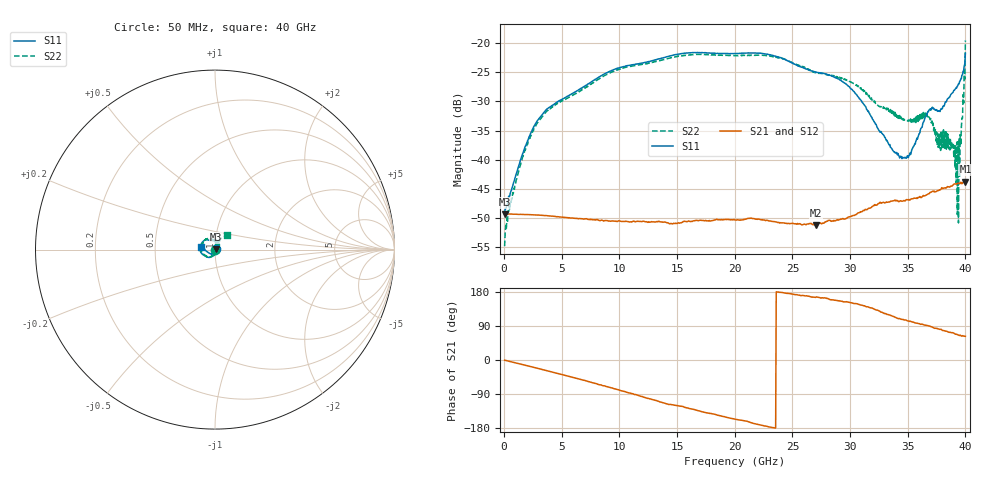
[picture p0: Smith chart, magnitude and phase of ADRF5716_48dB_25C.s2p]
! Device: ADRF5716
! Description: 30GHz 2-Bit Digital Attenuator
! Frequency: 100 MHz – 30 GHz
! Ports:
! ATTIN  = Port 1
! ATTOUT = Port 2
! State: 48 dB Attenuation selected
! Supply Voltage:
! VDD  =  +3.30 Volts
! VSS  =  -3.30 Volts
! Control Voltages:
! D5 = 3.3V, D6 = 3.3V
! Temperature = +25 C
! Data: Data was collected using a calibrated network analyzer.
!  The reference plane is the package pins of ADRF5716 switch.
! Note: Analog Devices supplies this data as a sample of measured data for this product.
!  Your particular data for this product may vary.
!  Analog Devices reserves the right to change this data at anytime
# HZ S DB R 50
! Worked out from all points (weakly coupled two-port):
!   800 points, 50 MHz to 40 GHz, reference 50 ohm
!   highest |S21| = -43.75 dB at 40 GHz (marker M1); lowest = -51.2 dB at 27.05 GHz (marker M2)
!   lowest |S11| = -49.4 dB at 50 MHz (marker M3), VSWR 1.01, Z = 50.3 + j0.089 ohm
!   |S11| at or under -10 dB: start of sweep to end of sweep
!   |S22| runs from -54.8 to -19.6 dB; largest |S21 - S12| = 0
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5e7  -49.36 15.0  -49.30 -0.6  -49.30 -0.6  -54.85 -1.6
5.5e8  -45.81 -2.9  -49.35 -4.2  -49.35 -4.2  -47.32 1.6
1.3e9  -40.91 -23.8  -49.40 -9.8  -49.40 -9.8  -41.75 -25.4
2.6e9  -34.27 -58.9  -49.47 -19.6  -49.47 -19.6  -34.58 -60.7
3.85e9  -31.12 -85.4  -49.64 -29.2  -49.64 -29.2  -31.38 -87.8
6.75e9  -27.67 -112.6  -50.15 -52.1  -50.15 -52.1  -28.07 -115.0
9.65e9  -24.43 -134.4  -50.55 -76.2  -50.55 -76.2  -24.68 -136.8
1.34e10  -22.71 -158.0  -50.56 -108.9  -50.56 -108.9  -23.03 -162.0
2.005e10  -21.78 162.1  -50.35 -156.4  -50.35 -156.4  -22.12 155.0
2.34e10  -22.19 138.4  -50.64 -178.8  -50.64 -178.8  -22.29 130.5
2.67e10  -24.79 119.0  -51.09 165.6  -51.09 165.6  -24.91 104.4
2.705e10  -24.98 117.1  -51.24 165.9  -51.24 165.9  -25.02 103.5
3e10  -27.69 85.7  -49.78 151.4  -49.78 151.4  -26.60 72.9
3.335e10  -37.33 38.9  -47.27 119.3  -47.27 119.3  -31.70 23.6
3.44e10  -39.43 6.0  -47.06 107.6  -47.06 107.6  -32.65 5.6
3.505e10  -39.65 -23.0  -46.89 103.0  -46.89 103.0  -33.20 -10.7
3.675e10  -31.74 -92.9  -45.91 90.8  -45.91 90.8  -32.31 -56.7
3.765e10  -31.62 -124.4  -45.31 82.1  -45.31 82.1  -37.89 -81.4
3.885e10  -28.58 -146.2  -44.54 72.0  -44.54 72.0  -37.74 -141.6
3.93e10  -27.40 -159.4  -44.10 67.0  -44.10 67.0  -49.41 -154.0
3.95e10  -26.56 -165.7  -44.16 64.6  -44.16 64.6  -42.85 93.8
4e10  -21.75 168.4  -43.75 62.6  -43.75 62.6  -19.55 50.9
